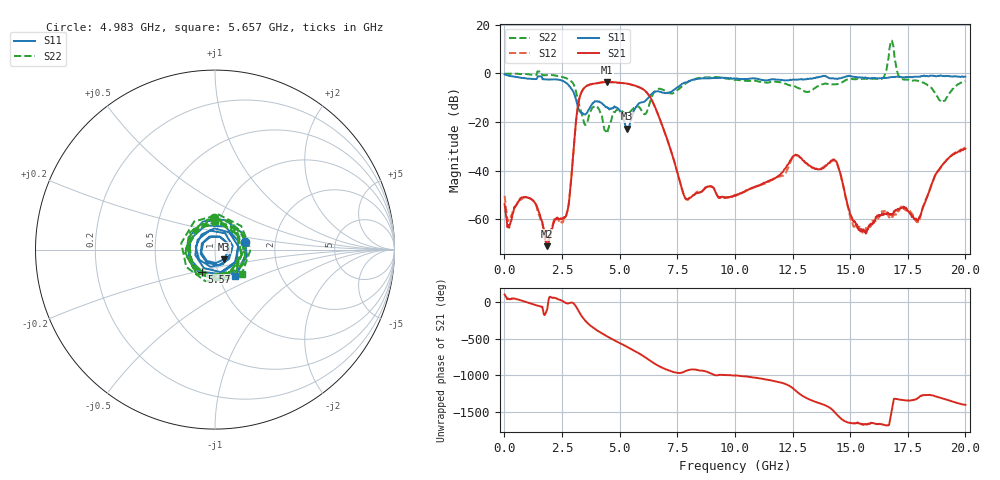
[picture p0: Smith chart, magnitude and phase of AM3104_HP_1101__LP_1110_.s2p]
!Created with skrf (http://scikit-rf.org).
# Hz S RI R 50.0
!freq ReS11 ImS11 ReS21 ImS21 ReS12 ImS12 ReS22 ImS22
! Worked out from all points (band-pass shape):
!   1601 points, 10 MHz to 20 GHz, reference 50 ohm
!   highest |S21| = -3.45 dB at 4.458 GHz (marker M1); lowest = -71.1 dB at 1.859 GHz (marker M2)
!   |S21| within 3 dB of the highest: 3.42 GHz to 6.012 GHz (2.591 GHz wide, 54.9 % of centre)
!   lowest |S11| = -22.7 dB at 5.332 GHz (marker M3), VSWR 1.16, Z = 54.8 - j5.98 ohm
!   |S11| at or under -10 dB: 3.087 GHz to 6.24 GHz (3.153 GHz wide, 67.6 % of centre)
!   |S22| runs from -24.7 to 13.6 dB; largest |S21 - S12| = 0.076
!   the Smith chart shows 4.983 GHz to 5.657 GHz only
!   S11 on the Smith chart (normalised r, x): 4.983 GHz: 1.40, +0.13; 5.57 GHz: 0.84, -0.21; 5.657 GHz: 1.19, -0.37
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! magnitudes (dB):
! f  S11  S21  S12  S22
! 10 MHz  -0.4  -53.8  -50.3  0.0
! 1.184 GHz  -2.2  -51.8  -51.9  -0.5
! 1.859 GHz  -2.5  -71.1  -68.9  -0.6
! 2.721 GHz  -4.2  -57.2  -56.9  -2.1
! 3.346 GHz  -16.2  -7.7  -7.7  -16.2
! 4.458 GHz  -13.9  -3.5  -3.5  -24.7
! 4.983 GHz  -15.2  -3.8  -3.8  -15.1
! 5.332 GHz  -22.7  -4.2  -4.2  -16.6
! 5.57 GHz  -16.8  -4.7  -4.7  -14.7
! 5.657 GHz  -14.6  -5.0  -5.0  -13.9
! 6.682 GHz  -7.3  -17.2  -17.2  -6.3
! 7.881 GHz  -3.7  -51.6  -51.6  -4.0
! 10.01 GHz  -2.2  -50.3  -50.3  -2.7
! 12.6 GHz  -2.6  -33.6  -33.6  -5.3
! 13.34 GHz  -2.2  -38.7  -38.6  -6.9
! 14.37 GHz  -2.1  -36.0  -36.3  -4.4
! 15.43 GHz  -1.6  -64.6  -63.4  -2.3
! 16.4 GHz  -1.9  -58.0  -57.2  -1.9
! 16.68 GHz  -1.6  -57.9  -59.1  7.3
! 17.95 GHz  -1.3  -60.2  -60.6  -3.0
! 19.01 GHz  -1.0  -37.6  -37.5  -11.7
! 20 GHz  -1.3  -31.0  -30.5  -3.1
